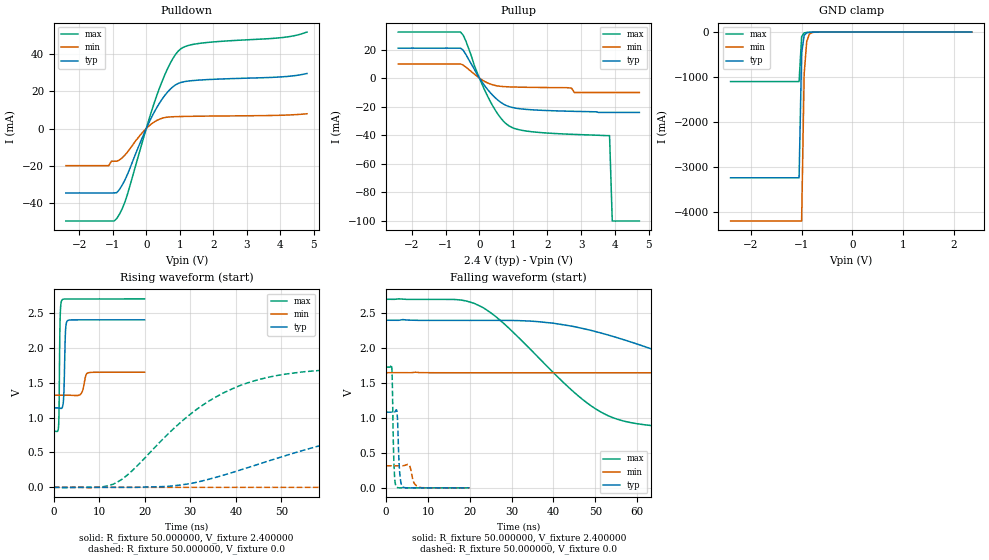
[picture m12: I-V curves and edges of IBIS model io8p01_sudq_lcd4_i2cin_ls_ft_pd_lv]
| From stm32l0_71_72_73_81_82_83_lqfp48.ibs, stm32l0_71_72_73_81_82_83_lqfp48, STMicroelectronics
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|   Model io8p01_sudq_lcd4_i2cin_ls_ft_pd_lv
[Model]  io8p01_sudq_lcd4_i2cin_ls_ft_pd_lv
Model_type I/O
Polarity   Non-Inverting
Enable   Active-Low
Vinl =   0.720000V
Vinh =   1.680000V
Vmeas =  1.200000V
Cref =   50.000000pF
Rref =   100.000000M
Vref =   0.0V
C_comp   2.470900pF   2.435200pF   2.490500pF
[Temperature Range]   25.000000   0.105000k   -40.000000
[Pullup Reference]   2.400000V   1.650000V   2.700000V
[Pulldown Reference]   0.0V   0.0V   0.0V
[POWER Clamp Reference]   2.400000V   1.650000V   2.700000V
[GND Clamp Reference]   0.0V   0.0V   0.0V
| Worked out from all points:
|   slope of the pulldown table from 0 to 0.36 V, typ, clamps not added: 28.5 ohm
|   slope of the pullup table from 0 to 0.36 V, typ, clamps not added: 32.2 ohm
|   GND clamp passes 1 mA (typ) near -0.64 V on its own axis
|   rising waveform, R_fixture 50.000000, V_fixture 2.400000: 20-80 % time 282ps typ, 635ps min, 192ps max; typ from 1.14 V to 2.4 V
|   rising waveform, R_fixture 50.000000, V_fixture 0.0: 20-80 % time 39.6ns typ, 106ns min, 19.4ns max; typ from 0 V to 1.08 V
|   falling waveform, R_fixture 50.000000, V_fixture 2.400000: 20-80 % time 40.8ns typ, 106ns min, 20.1ns max; typ from 2.4 V to 1.14 V
|   falling waveform, R_fixture 50.000000, V_fixture 0.0: 20-80 % time 455ps typ, 827ps min, 357ps max; typ from 1.08 V to 0 V
[Pulldown]
|Voltage   I(typ)   I(min)   I(max)
-2.4V     -34.7mA    -20mA      -49.82mA
-1.12V    -34.7mA    -20mA      -49.82mA
-1.04V    -34.7mA    -17.6mA    -49.82mA
-880mV    -34.55mA   -17.6mA    -48.46mA
-560mV    -24.65mA   -12.68mA   -35.33mA
0V        224fA      0A         16fA
400mV     13.84mA    5.066mA    22.03mA
720mV     21.25mA    6.254mA    35.26mA
1.04V     24.83mA    6.464mA    43.03mA
1.6V      26.11mA    6.627mA    45.88mA
4V        27.76mA    7.125mA    48.88mA
4.8V      29.64mA    7.94mA     51.96mA
[Pullup]
|Voltage   I(typ)   I(min)   I(max)
-2.4V     21.06mA    9.987mA    32.34mA
-560mV    21.06mA    9.987mA    32.34mA
-400mV    16.53mA    7.734mA    25.89mA
-80mV     3.011mA    1.498mA    4.671mA
320mV     -10.16mA   -4.078mA   -16.34mA
640mV     -17.08mA   -5.718mA   -28.28mA
960mV     -20.45mA   -6.129mA   -34.5mA
1.76V     -22.39mA   -6.471mA   -37.97mA
2.8V      -23.2mA    -10mA      -39.35mA
3.84V     -24mA      -10mA      -40.2mA
3.92V     -24mA      -10mA      -100mA
4.72V     -24mA      -10mA      -100mA
[GND_clamp]
|Voltage   I(typ)   I(min)   I(max)
-2.4V     -3.237A    -4.197A    -1.1A
-1.05V    -3.237A    -4.197A    -1.1A
-1V       -475.5mA   -4.197A    -104.1mA
-950mV    -76.09mA   -935.1mA   -18.45mA
-900mV    -16.59mA   -212.6mA   -9.272mA
-850mV    -6.633mA   -50.89mA   -6.773mA
-800mV    -4.105mA   -13.86mA   -5.003mA
-650mV    -1.082mA   -1.227mA   -1.183mA
2.35V     52.69uA    50.02uA    36.84uA
[POWER_clamp]
|Voltage   I(typ)   I(min)   I(max)
-2.4V     0A         0A         0A
0V        0A         0A         0A
[Ramp]
| variable   typ   min   max
dV/dt_r  0.65004/39.51594n   0.18943/0.10635u   1.03746/19.38110n
dV/dt_f  0.75702/40.79785n   0.19512/0.10583u   1.13800/20.05849n
R_load = 50.000000
[Rising Waveform]
R_fixture= 50.000000
V_fixture= 2.400000
V_fixture_min= 1.650000
V_fixture_max= 2.700000
|time   V(typ)   V(min)   V(max)
0s        1.137V     1.32V      802.9mV
1.041ns   1.137V     1.32V      870.2mV
1.161ns   1.136V     1.32V      1.189V
1.361ns   1.133V     1.32V      2.354V
1.762ns   1.134V     1.32V      2.68V
2.202ns   1.341V     1.32V      2.696V
2.603ns   2.275V     1.32V      2.697V
2.963ns   2.383V     1.32V      2.698V
7.608ns   2.399V     1.641V     2.698V
19.94ns   2.399V     1.649V     2.7V
[Rising Waveform]
R_fixture= 50.000000
V_fixture= 0.0
V_fixture_min= 0.0
V_fixture_max= 0.0
|time   V(typ)   V(min)   V(max)
0s        1.262nV    6.192nV    1.046nV
14.01ns   -210.4uV   -46.19uV   76.8mV
30.03ns   54.59mV    -45.9uV    1.049V
40.04ns   229mV      -45.98uV   1.434V
49.05ns   415.7mV    -39.05uV   1.601V
61.06ns   639.9mV    16.55uV    1.688V
87.09ns   930.8mV    1.188mV    1.725V
124.1ns   1.056V     41.68mV    1.729V
255.3ns   1.083V     267.1mV    1.729V
498.5ns   1.083V     316.1mV    1.729V
[Falling Waveform]
R_fixture= 50.000000
V_fixture= 2.400000
V_fixture_min= 1.650000
V_fixture_max= 2.700000
|time   V(typ)   V(min)   V(max)
0s        2.399V     1.649V     2.7V
21.02ns   2.397V     1.648V     2.642V
28.03ns   2.397V     1.648V     2.358V
50.05ns   2.237V     1.648V     1.131V
58.06ns   2.097V     1.648V     938.9mV
71.07ns   1.826V     1.648V     856.3mV
99.1ns    1.361V     1.647V     814.3mV
136.1ns   1.199V     1.633V     804.8mV
288.3ns   1.138V     1.378V     802.9mV
498.5ns   1.137V     1.32V      802.9mV
[Falling Waveform]
R_fixture= 50.000000
V_fixture= 0.0
V_fixture_min= 0.0
V_fixture_max= 0.0
|time   V(typ)   V(min)   V(max)
0s        1.083V     316.1mV    1.729V
1.321ns   1.083V     316.1mV    1.745V
1.441ns   1.083V     316.1mV    1.583V
1.882ns   1.083V     316.1mV    322.2mV
2.442ns   1.117V     316.1mV    17.08mV
2.683ns   1.012V     316.1mV    5.077mV
3.203ns   247.5mV    315.9mV    506.7uV
3.804ns   20.76mV    315.6mV    181.5uV
7.928ns   40.13uV    7.533mV    -1.669uV
19.94ns   1.262nV    6.192nV    1.046nV
